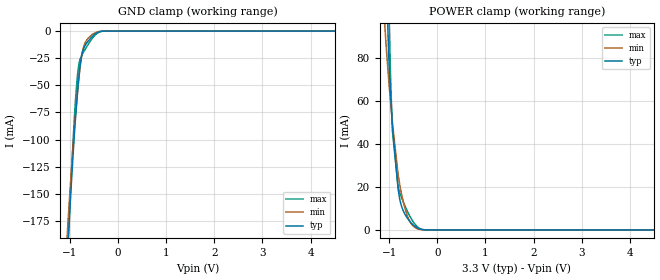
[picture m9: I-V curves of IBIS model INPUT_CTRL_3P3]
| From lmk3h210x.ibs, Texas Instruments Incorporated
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[Model]   INPUT_CTRL_3P3
Model_type   Input
Vinl = 0.65
Vinh = 1.15
|   typ   min   max
C_comp   0.7pF   0.5pF   0.9pF
[Voltage Range]   3.3   3.135   3.465
[Temperature Range]   45   125   -40
[Power Clamp Reference]   3.3   3.135   3.465
[GND Clamp Reference]   0   0   0
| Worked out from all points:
|   GND clamp passes 1 mA (typ) near -0.41 V on its own axis
|   POWER clamp passes 1 mA (typ) near -0.42 V on its own axis
[GND Clamp]
|   Voltage   I(typ)   I(min)   I(max)
-3.3V     -2.474A    -2.191A    -2.782A
-1.132V   -277.9mA   -243.6mA   -280mA
-1.043V   -198.1mA   -176.1mA   -194.8mA
-1.033V   -189.6mA   -169mA     -185.7mA
-1.013V   -173mA     -155.2mA   -167.6mA
-904.2mV  -91.28mA   -86.97mA   -75.43mA
-844.8mV  -56.1mA    -55.89mA   -39.89mA
-815.1mV  -41.69mA   -42.5mA    -30.02mA
-765.6mV  -24.25mA   -24.86mA   -23.17mA
-706.2mV  -14.74mA   -12.92mA   -18.37mA
-468.6mV  -2.382mA   -1.374mA   -3.243mA
6.6V      0A         0A         0A
[POWER Clamp]
|   Voltage   I(typ)   I(min)   I(max)
-3.3V     4.358A     3.47A      5.491A
-1.102V   157.7mA    98.45mA    260.4mA
-1.063V   117.7mA    84.69mA    188.7mA
-1.013V   82.15mA    70.06mA    113.5mA
-1.003V   76.72mA    67.34mA    101.2mA
-973.5mV  62.88mA    59.5mA     70.99mA
-933.9mV  48.27mA    49.68mA    45.88mA
-815.1mV  18.76mA    25.75mA    19.77mA
-745.8mV  11.11mA    16.79mA    15.13mA
-617.1mV  5.305mA    6.137mA    8.372mA
-419.1mV  967.2uA    633.2uA    1.571mA
6.6V      0A         0A         0A
